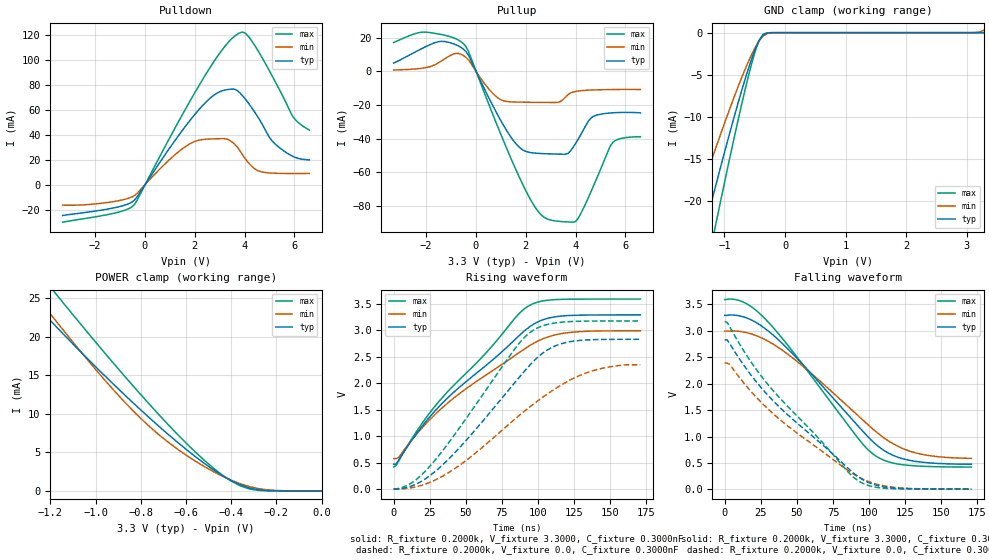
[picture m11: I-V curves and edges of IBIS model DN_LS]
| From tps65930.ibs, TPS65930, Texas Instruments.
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|   Model DN_LS
[Model]  DN_LS
Model_type 3-state
Polarity   Inverting
Enable   Active-Low
|Vinl =   1.1550V
|Vinh =   2.1450V
Vmeas =  1.6500V
Cref =   0.3000nF
Rref =   100.0000M
Vref =   0.0V
C_comp   6.1523pF   6.1128pF   6.1708pF
[Temperature Range]   25.0000   0.1250k   -40.0000
[Pullup Reference]   3.3000V   3.0000V   3.6000V
[Pulldown Reference]   0.0V   0.0V   0.0V
[POWER Clamp Reference]   3.3000V   3.0000V   3.6000V
[GND Clamp Reference]   0.0V   0.0V   0.0V
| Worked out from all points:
|   slope of the pulldown table from 0 to 0.495 V, typ, clamps not added: 33.1 ohm
|   slope of the pullup table from 0 to 0.495 V, typ, clamps not added: 32.5 ohm
|   GND clamp passes 1 mA (typ) near -0.43 V on its own axis
|   POWER clamp passes 1 mA (typ) near -0.38 V on its own axis
|   rising waveform, R_fixture 0.2000k, V_fixture 3.3000, C_fixture 0.3000nF: 20-80 % time 64.7ns typ, 66.6ns min, 60.9ns max; typ from 0.474 V to 3.29 V
|   rising waveform, R_fixture 0.2000k, V_fixture 0.0, C_fixture 0.3000nF: 20-80 % time 53.8ns typ, 64.3ns min, 49.7ns max; typ from 0.003 V to 2.83 V
|   falling waveform, R_fixture 0.2000k, V_fixture 3.3000, C_fixture 0.3000nF: 20-80 % time 56.6ns typ, 59.9ns min, 53ns max; typ from 3.29 V to 0.477 V
|   falling waveform, R_fixture 0.2000k, V_fixture 0.0, C_fixture 0.3000nF: 20-80 % time 63.3ns typ, 62.9ns min, 60.6ns max; typ from 2.83 V to 0.007 V
[Pulldown]
|Voltage   I(typ)   I(min)   I(max)
-3.3V     -24.66mA   -16.41mA   -30.04mA
-1.1V     -17.95mA   -13mA      -22.2mA
-400mV    -12.07mA   -8.474mA   -15.4mA
1.1V      32.31mA    22.07mA    41.3mA
2V        56.12mA    34.56mA    73.51mA
3V        74.4mA     36.82mA    105.2mA
3.4V      76.38mA    35.58mA    115.2mA
3.8V      73.84mA    27.66mA    121.5mA
4.2V      64.12mA    16.57mA    117.6mA
5.2V      33.12mA    9.179mA    83.64mA
6V        22.07mA    8.949mA    52.91mA
6.6V      19.86mA    9.006mA    43.68mA
[Pullup]
|Voltage   I(typ)   I(min)   I(max)
-3.3V     4.986mA    892.9uA    17.22mA
-1.5V     17.71mA    5.182mA    22.3mA
-500mV    13.29mA    9.474mA    16.55mA
800mV     -23.75mA   -14.72mA   -30.01mA
1.6V      -42.83mA   -18.18mA   -58.24mA
2.4V      -48.58mA   -18.36mA   -81.24mA
2.9V      -48.96mA   -18.42mA   -87.9mA
3.7V      -48.66mA   -13.73mA   -89.49mA
4V        -42.83mA   -11.87mA   -89.19mA
4.6V      -27.88mA   -11.04mA   -72.1mA
5.5V      -24.57mA   -10.73mA   -42.09mA
6.6V      -24.6mA    -10.73mA   -38.85mA
[GND_clamp]
|Voltage   I(typ)   I(min)   I(max)
-3.3V     -81.85mA   -63mA      -101.5mA
-1.62V    -31.7mA    -23.93mA   -39.66mA
-1.55V    -29.68mA   -22.39mA   -37.14mA
-1.34V    -23.66mA   -17.84mA   -29.65mA
-1.27V    -21.68mA   -16.35mA   -27.18mA
-1.13V    -17.78mA   -13.42mA   -22.3mA
-780mV    -8.466mA   -6.506mA   -10.53mA
-570mV    -3.5mA     -2.877mA   -4.17mA
-430mV    -952.3uA   -990.8uA   -936.3uA
-360mV    -254.5uA   -387.4uA   -175.3uA
-150mV    -159.5nA   -2.336uA   -11.79nA
3.28V     -1.065nA   287.8uA    719.4fA
[POWER_clamp]
|Voltage   I(typ)   I(min)   I(max)
-3.28V    107.5mA    105.3mA    115.4mA
-1.32V    25.97mA    27.48mA    30.86mA
-1.28V    24.66mA    25.97mA    29.39mA
-1.24V    23.38mA    24.47mA    27.92mA
-1.16V    20.89mA    21.5mA     25.02mA
-920mV    13.83mA    13.09mA    16.55mA
-760mV    9.439mA    8.315mA    11.19mA
-600mV    5.408mA    4.656mA    6.228mA
-440mV    2.013mA    1.929mA    2.07mA
-320mV    385.2uA    564.3uA    258.4uA
-200mV    11.92uA    55.37uA    2.562uA
0V        2.348nA    59.16nA    498.2pA
[Ramp]
| variable   typ   min   max
dV/dt_r  0.1695/12.9594n   94.0119m/12.3471n   0.2654/13.6266n
dV/dt_f  0.2120/15.0408n   0.1440/14.2087n   0.2860/14.9171n
R_load = 50.0000
[Rising Waveform]
R_fixture= 0.2000k
V_fixture= 3.3000
V_fixture_min= 3.0000
V_fixture_max= 3.6000
C_fixture= 0.3000nF
|time   V(typ)   V(min)   V(max)
0s        474.5mV    579.1mV    422.8mV
3.434ns   551.2mV    600.9mV    533.6mV
18.89ns   1.162V     1.135V     1.215V
34.34ns   1.643V     1.557V     1.752V
61.82ns   2.291V     2.118V     2.512V
85.86ns   2.874V     2.562V     3.288V
92.73ns   3.039V     2.688V     3.449V
104.7ns   3.212V     2.855V     3.562V
118.5ns   3.275V     2.948V     3.586V
170.8ns   3.292V     2.993V     3.59V
[Rising Waveform]
R_fixture= 0.2000k
V_fixture= 0.0
V_fixture_min= 0.0
V_fixture_max= 0.0
C_fixture= 0.3000nF
|time   V(typ)   V(min)   V(max)
0s        3.146mV    3.904mV    3.322mV
15.45ns   98.36mV    47.45mV    181.4mV
32.63ns   430.2mV    229.9mV    684.7mV
53.23ns   1.019V     610.5mV    1.456V
84.14ns   2.022V     1.33V      2.659V
96.16ns   2.398V     1.596V     2.993V
108.2ns   2.658V     1.833V     3.122V
120.2ns   2.776V     2.034V     3.162V
144.2ns   2.828V     2.283V     3.176V
170.8ns   2.831V     2.351V     3.177V
[Falling Waveform]
R_fixture= 0.2000k
V_fixture= 3.3000
V_fixture_min= 3.0000
V_fixture_max= 3.6000
C_fixture= 0.3000nF
|time   V(typ)   V(min)   V(max)
0s        3.292V     2.993V     3.59V
13.74ns   3.257V     2.974V     3.533V
29.19ns   3.017V     2.815V     3.192V
53.23ns   2.387V     2.351V     2.39V
92.73ns   1.188V     1.385V     953.6mV
104.7ns   851.2mV    1.092V     630.5mV
116.8ns   642.3mV    860.5mV    497.4mV
130.5ns   537.7mV    704.2mV    448.6mV
147.7ns   491.4mV    619.2mV    429.3mV
170.8ns   476.9mV    588.4mV    423.4mV
[Falling Waveform]
R_fixture= 0.2000k
V_fixture= 0.0
V_fixture_min= 0.0
V_fixture_max= 0.0
C_fixture= 0.3000nF
|time   V(typ)   V(min)   V(max)
0s        2.831V     2.39V      3.177V
3.434ns   2.76V      2.364V     3.077V
17.17ns   2.201V     1.885V     2.454V
30.91ns   1.752V     1.498V     1.953V
46.36ns   1.344V     1.143V     1.493V
85.86ns   388.5mV    349mV      317.4mV
92.73ns   235.7mV    233.7mV    159.4mV
103ns     95.54mV    116.6mV    50.22mV
113.3ns   36.75mV    54.8mV     18.21mV
170.8ns   6.586mV    5.153mV    7.91mV
